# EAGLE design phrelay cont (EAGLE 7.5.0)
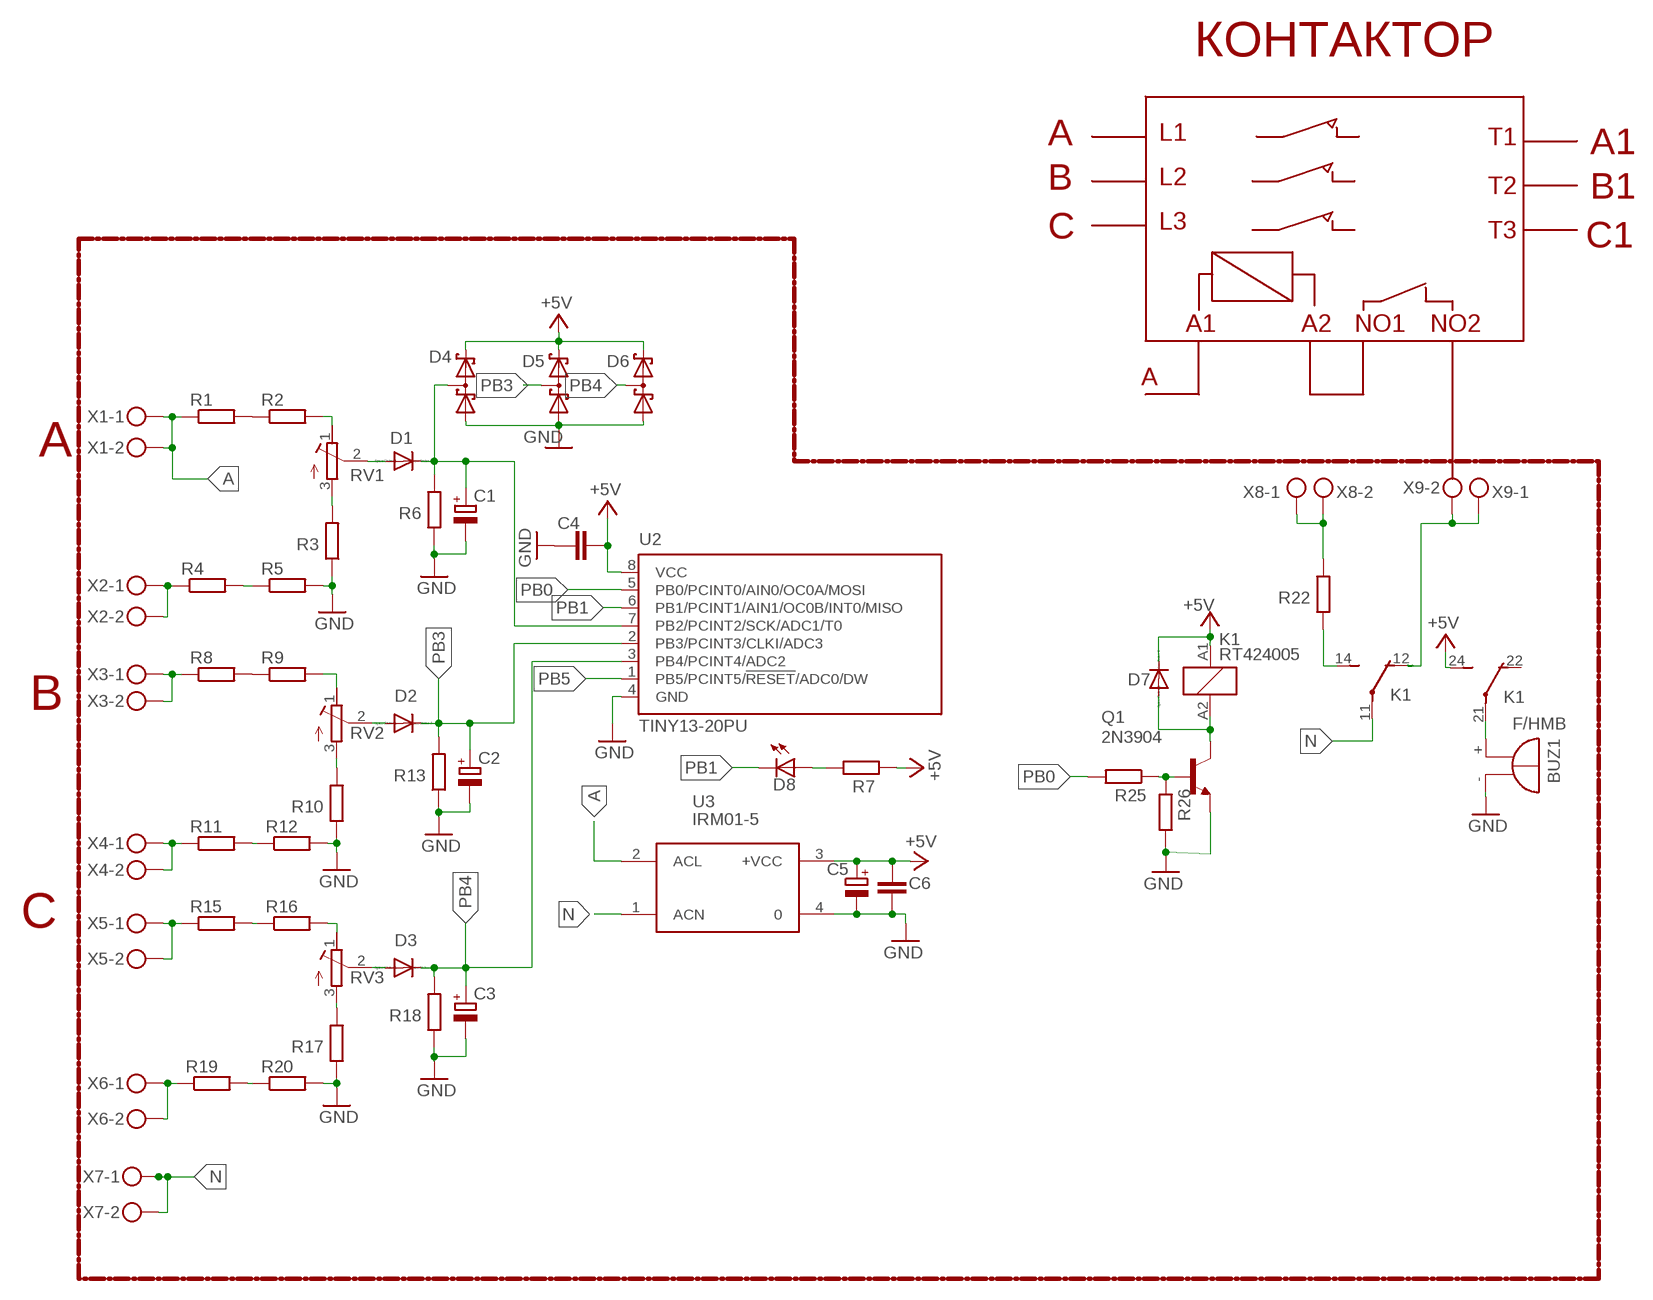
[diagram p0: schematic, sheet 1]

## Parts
BUZ1  F/HMB  [F/HMB]
C1  CPOL-EUE2-5  [E2-5]
C2  CPOL-EUE2-5  [E2-5]
C3  CPOL-EUE2-5  [E2-5]
C4  C-EUC1206  [C1206]
C5  CPOL-EUE2-5  [E2-5]
C6  C-EUC1206  [C1206]
D1  1N4004  [DO41-10]
D2  1N4004  [DO41-10]
D3  1N4004  [DO41-10]
D4  BAT54S  [SOT23]
D5  BAT54S  [SOT23]
D6  BAT54S  [SOT23]
D7  1N4004  [DO41-10]
D8  LED5MM  [LED5MM]
K1  RT424005  [RT2C/O]
Q1  2N3904  [TO92]
R1  R-EU_0414/15  [0414/15]
R2  R-EU_0414/15  [0414/15]
R3  R-EU_0309/12  [0309/12]
R4  R-EU_0414/15  [0414/15]
R5  R-EU_0414/15  [0414/15]
R6  R-EU_R1206  [R1206]
R7  R-EU_R1206  [R1206]
R8  R-EU_0414/15  [0414/15]
R9  R-EU_0414/15  [0414/15]
R10  R-EU_0309/12  [0309/12]
R11  R-EU_0414/15  [0414/15]
R12  R-EU_0414/15  [0414/15]
R13  R-EU_R1206  [R1206]
R15  R-EU_0414/15  [0414/15]
R16  R-EU_0414/15  [0414/15]
R17  R-EU_0309/12  [0309/12]
R18  R-EU_R1206  [R1206]
R19  R-EU_0414/15  [0414/15]
R20  R-EU_0414/15  [0414/15]
R22  R-EU_0309/12  [0309/12]
R25  R-EU_R1206  [R1206]
R26  R-EU_R1206  [R1206]
RV1  R-TRIMM-3386-F  [R-TRIMM-3386F]
RV2  R-TRIMM-3386-F  [R-TRIMM-3386F]
RV3  R-TRIMM-3386-F  [R-TRIMM-3386F]
U2  TINY13-20PU  [DIL08]
U3  IRM01-5  IRM05-2  [IRM05-2]
X1  MKDSN1,5/2-5,08  [MKDSN1,5/2-5,08]
X2  MKDSN1,5/2-5,08  [MKDSN1,5/2-5,08]
X3  MKDSN1,5/2-5,08  [MKDSN1,5/2-5,08]
X4  MKDSN1,5/2-5,08  [MKDSN1,5/2-5,08]
X5  MKDSN1,5/2-5,08  [MKDSN1,5/2-5,08]
X6  MKDSN1,5/2-5,08  [MKDSN1,5/2-5,08]
X7  MKDSN1,5/2-5,08  [MKDSN1,5/2-5,08]
X8  MKDSN1,5/2-5,08  [MKDSN1,5/2-5,08]
X9  MKDSN1,5/2-5,08  [MKDSN1,5/2-5,08]

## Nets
+5V: C4.2 C5.+ C6.2 D4.2(C2) D5.2(C2) D6.2(C2) D7.C K1.24(3:S) K1.A1 R7.1 U2.8(VCC) U3.3(+VCC)
A: R1.1 U3.2(ACL) X1.1 X1.2
GND: BUZ1.- C1.- C2.- C3.- C4.1 C5.- C6.1 D4.1(A1) D5.1(A1) D6.1(A1) Q1.3(E) R3.1 R5.2 R6.1 R10.1 R12.2 R13.1 R17.1 R18.1 R20.2 R26.2 U2.4(GND) U3.4
N: K1.11(2:P) U3.1(ACN) X7.1 X7.2
N$1: R8.2 R9.1
N$2: R2.2 RV1.1(A)
N$3: R1.2 R2.1
N$4: R3.2 RV1.3(E)
N$5: D1.A RV1.2(S)
N$6: C1.+ D1.C D4.3(C1A2) R6.2 U2.7(PB2/PCINT2/SCK/ADC1/T0)
N$7: R4.1 X2.1 X2.2
N$8: R4.2 R5.1
N$9: R19.1 X6.1 X6.2
N$10: R9.2 RV2.1(A)
N$11: R10.2 RV2.3(E)
N$12: D8.A R7.2
N$13: Q1.2(B) R25.1 R26.1
N$14: R11.2 R12.1
N$15: R8.1 X3.1 X3.2
N$16: R17.2 RV3.3(E)
N$17: R16.2 RV3.1(A)
N$18: R15.2 R16.1
N$19: D2.A RV2.2(S)
N$20: D3.A RV3.2(S)
N$21: D7.A K1.A2 Q1.1(C)
N$22: R11.1 X4.1 X4.2
N$23: R19.2 R20.1
N$24: R15.1 X5.1 X5.2
N$25: BUZ1.+ K1.21(3:P)
N$26: R22.2 X8.1 X8.2
N$27: K1.12(2:O) X9.1 X9.2
N$29: K1.14(2:S) R22.1
PB0: R25.2 U2.5(PB0/PCINT0/AIN0/OC0A/MOSI)
PB1: D8.K(C) U2.6(PB1/PCINT1/AIN1/OC0B/INT0/MISO)
PB3: C2.+ D2.C D5.3(C1A2) R13.2 U2.2(PB3/PCINT3/CLKI/ADC3)
PB4: C3.+ D3.C D6.3(C1A2) R18.2 U2.3(PB4/PCINT4/ADC2)
PB5: U2.1(PB5/PCINT5/!RESET!/ADC0/DW)
Unconnected: K1.22(3:O)

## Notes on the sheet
- КОНТАКТОР
- A | L1 | T1
- A1
- B | L2
- T2 | B1
- L3
- C | T3 | C1
- A1 | A2 | NO1 | NO2
- А
- A
- B
- C

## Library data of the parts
BUZ1 = buzzer:F/HMB: BUZZER; OC_FARNELL: unknown; OC_NEWARK: unknown
C1-C3 C5 = rcl:CPOL-EU: POLARIZED CAPACITOR, European symbol
C4 C6 = rcl:C-EU: CAPACITOR, European symbol
D1-D3 D7 = diode:1N4004: DIODE
D4-D6 = diode:BAT54S: Schottky Diodes Pin connection corrected 2011-05-04 Source: Fairchild .. BAT54.pdf
D8 = led:LED: LED
K1 = relay:RT42?*: Power PCB Relay SCHRACK 2 pole 8 A, DC and AC-coil Source: http://www.schrack.com/.. 5842.pdf; MPN: RT424005; OC_FARNELL: 1629052; OC_NEWARK: 03P2425
Q1 = transistor:2N3904: NPN TRANSISTOR
R1-R13 R15-R20 R22 R25 R26 = rcl:R-EU_: RESISTOR, European symbol
RV1-RV3 = rcl:R-TRIMM-3386-F
U2 = atmel:TINY13: 8-bit AVR Microcontroller with 1K Bytes In-System Programmable Flash Source: http://www.atmel.com/dyn/resources/prod_documents/2535S.pdf; MPN: ATTINY13-20PU; OC_FARNELL: 9171550; OC_NEWARK: 96K6521
U3 = acdc:IRM05-2
X1-X9 = con-phoenix-508:MKDSN1,5/2-5,08: MKDSN 1,5/ 2-5,08 Printklemme

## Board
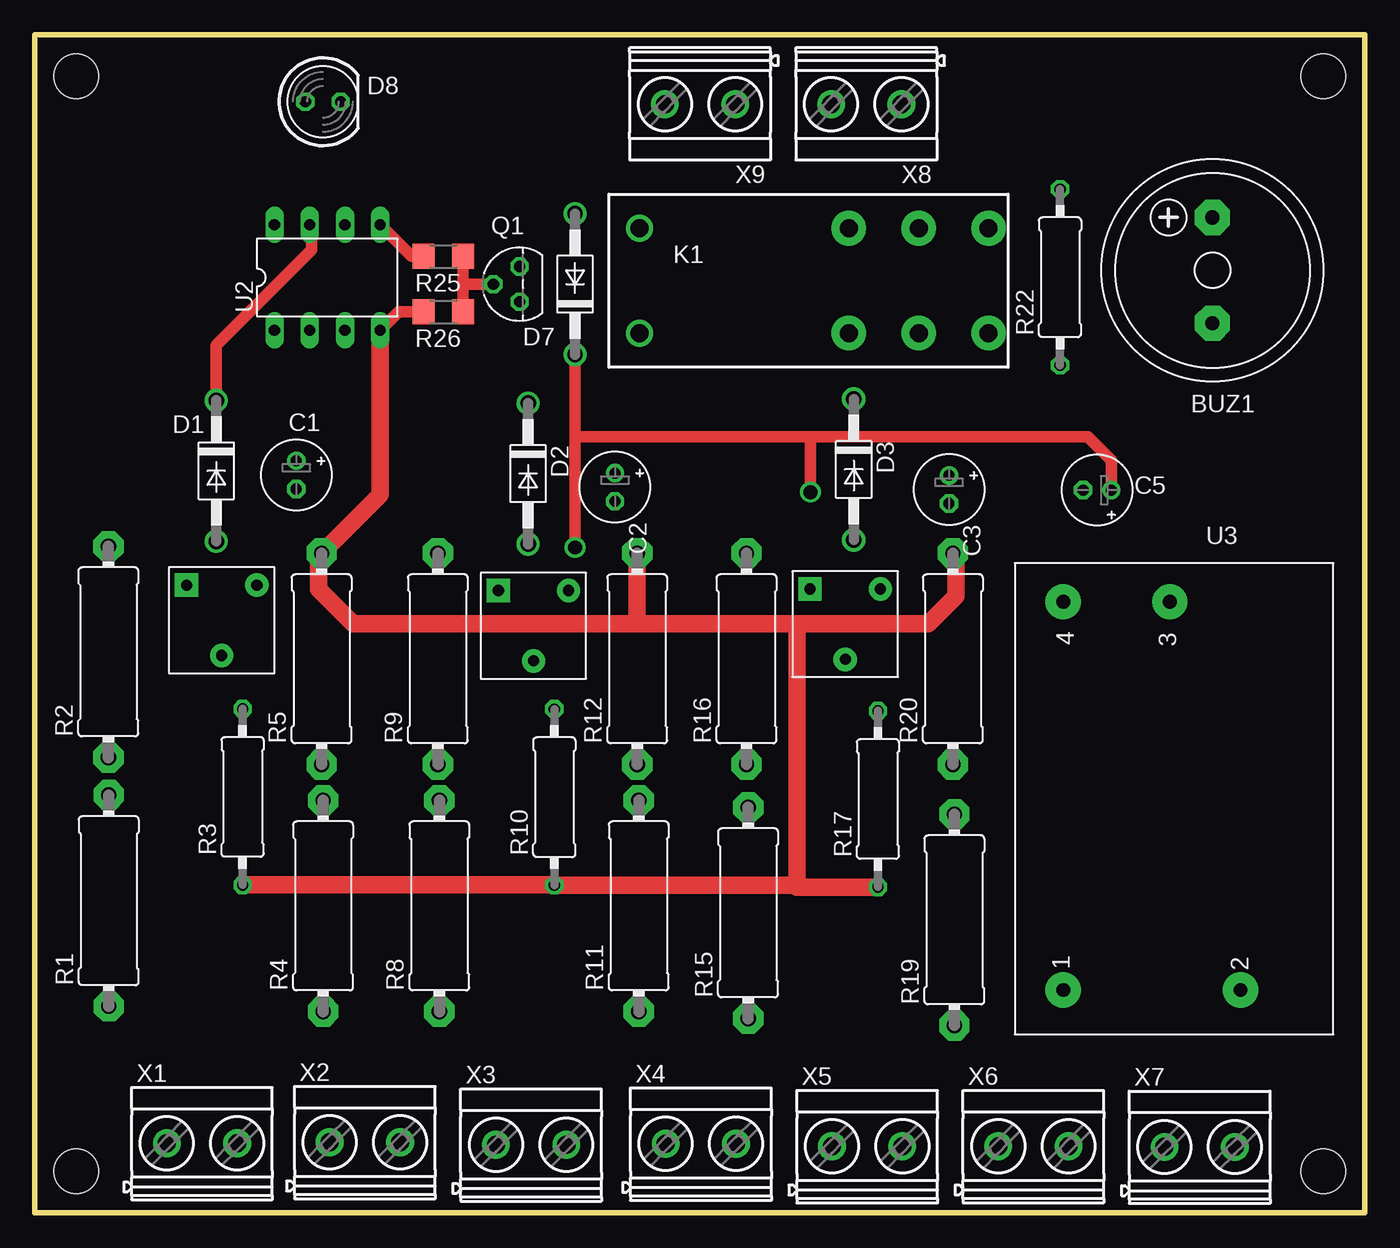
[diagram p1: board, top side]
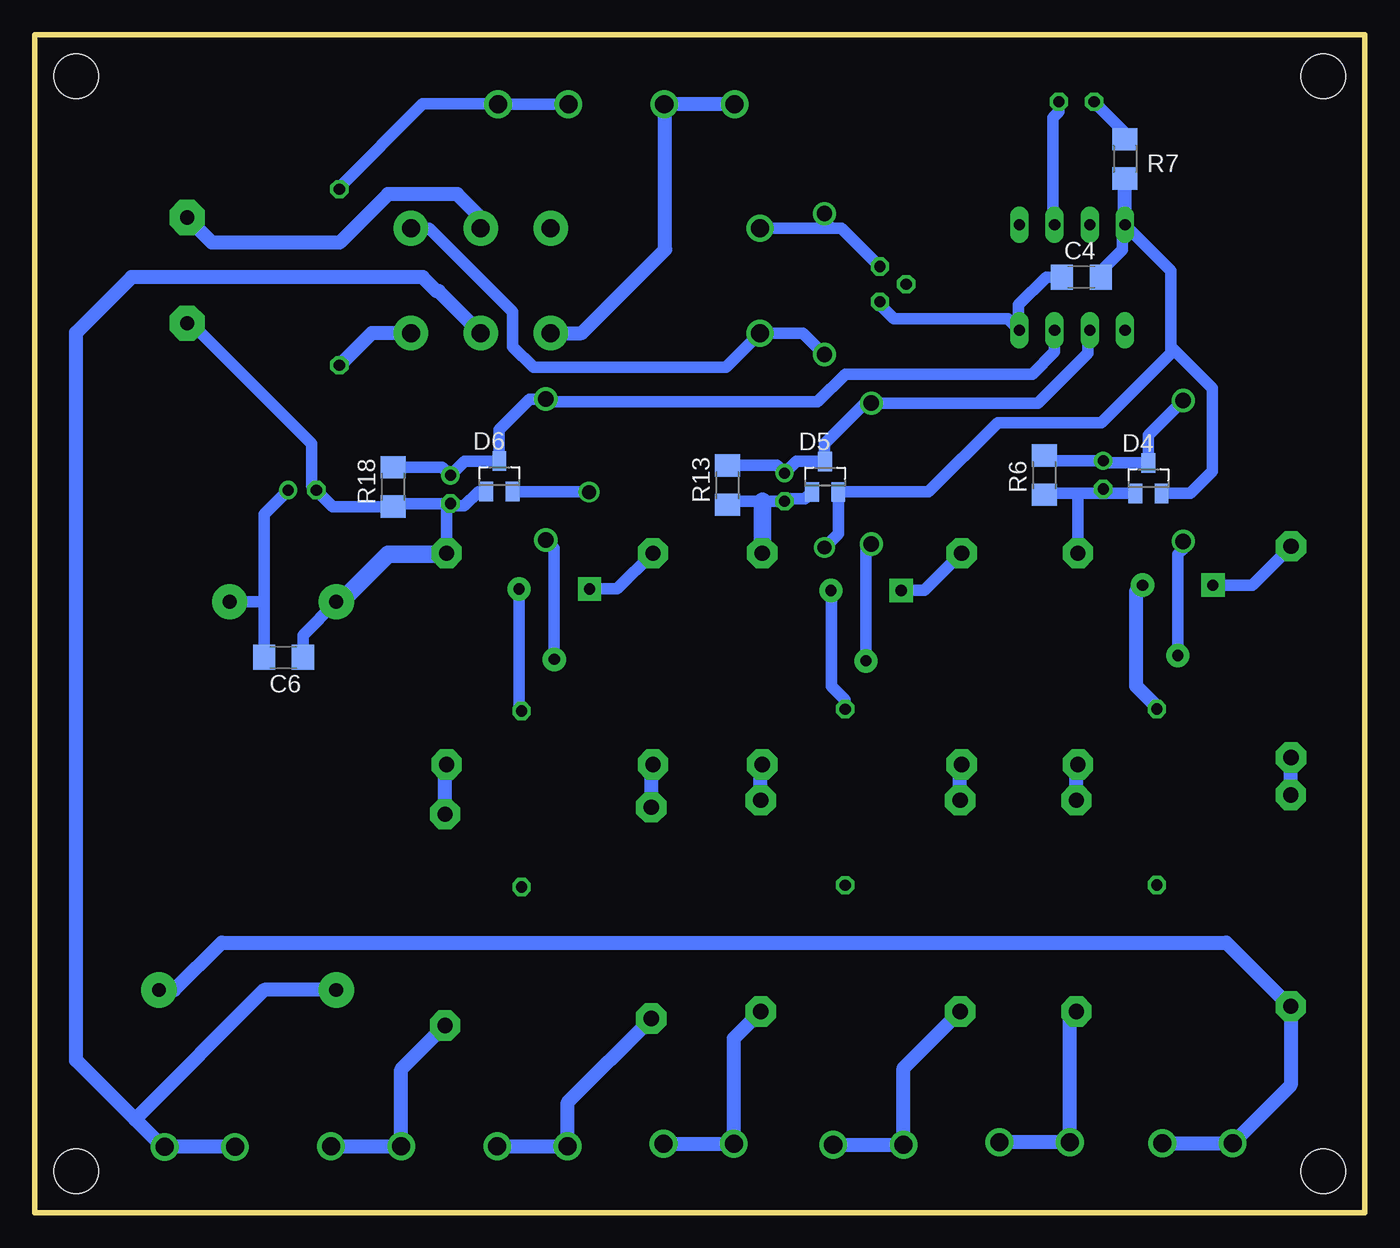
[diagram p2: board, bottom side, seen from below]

Size 96 x 85 mm. Coordinates in mm from the lower left corner, seen from the top.
Outline: 0,0 96,0 96,85 0,85 0,0
Copper layers (1*16): Top 0.035mm / dielectric 1.5mm / Bottom 0.035mm
Design rules "default": minimum track width 10mil, minimum drill 24mil, track to track 8mil, track to pad 8mil, pad to pad 8mil, via to via 8mil, smd to smd 8mil, copper to edge 40mil, drill to drill 8mil, minimum pad ring 10mil, minimum via ring 8mil, stop-mask expansion 4mil, vias tented up to drill 0mil, thermal gap 10mil
Holes 3.2 mm at 3,3 93,3 3,82 93,82

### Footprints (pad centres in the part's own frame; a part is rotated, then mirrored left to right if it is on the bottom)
F/HMB = drill 1.016 pad 2.54 octagon: + 3.81,0; - -3.81,0
E2-5 = drill 0.813 pad 1.27: + -1.016,0 | drill 0.813 pad 1.27 octagon: - 1.016,0
C1206 = smd 1.6 x 1.8: 1 -1.4,0; 2 1.4,0
DO41-10 = drill 1.118: A 5.08,0; C -5.08,0
SOT23 = smd 1 x 1.4: 1 -0.95,-1.1; 2 0.95,-1.1; 3 0,1.1
LED5MM = drill 0.813 octagon: A -1.27,0; K 1.27,0
RT2C/O = drill 1.3 pad 2.5: 11 7.56,-3.68; 12 2.52,-3.68; 14 12.6,-3.68; 21 7.56,3.88; 22 2.52,3.88; 24 12.6,3.88 | drill 1.3: A1 -12.6,-3.68; A2 -12.6,3.88
TO92 = drill 0.813 octagon: 1 1.27,0; 2 0,1.905; 3 -1.27,0
0414/15 = drill 1.1 pad 2.184 octagon: 1 -7.62,0; 2 7.62,0
0309/12 = drill 0.813 octagon: 1 -6.35,0; 2 6.35,0
R1206 = smd 1.6 x 1.803: 1 -1.422,0; 2 1.422,0
R-TRIMM-3386F = drill 0.8 pad 1.676 square: 1 0,0 | drill 0.8 pad 1.676: 2 5.08,2.54; 3 0,5.08
DIL08 = drill 0.813 long: 1 -3.81,-3.81; 2 -1.27,-3.81; 3 1.27,-3.81; 4 3.81,-3.81; 5 3.81,3.81; 6 1.27,3.81; 7 -1.27,3.81; 8 -3.81,3.81
IRM05-2 = drill 1 pad 2.54: 1 30.8,3.5; 2 30.8,16.3; 3 2.8,11.2; 4 2.8,3.5
MKDSN1,5/2-5,08 = drill 1.3 pad 2: 1 -2.561,0.025; 2 2.519,0.025

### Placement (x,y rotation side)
BUZ1  85,68 90 top
C1  18.88,53.24 270 top
C2  41.88,52.35 270 top
C3  65.99,52.19 270 top
C4  20.46,67.51 0 bottom
C5  76.69,52.14 180 top
C6  78.04,40.07 180 bottom
D1  13.11,53.53 270 top
D2  35.61,53.33 270 top
D3  59.11,53.63 270 top
D4  15.62,53 0 bottom
D5  38.96,53.11 0 bottom
D6  62.46,53.14 0 bottom
D7  39,67 90 top
D8  20.81,80.16 0 top
K1  56.24,67.15 0 top
Q1  35,67 90 top
R1  5.35,22.52 90 top
R2  5.32,40.47 90 top
R3  15.01,30.01 90 top
R4  20.82,22.14 90 top
R5  20.71,39.97 90 top
R6  23.14,53.22 90 bottom
R7  17.31,76.04 90 bottom
R8  29.21,22.14 90 top
R9  29.1,39.97 90 top
R10  37.51,29.99 90 top
R11  43.6,22.14 90 top
R12  43.49,39.97 90 top
R13  46,52.5 90 bottom
R15  51.49,21.64 90 top
R16  51.38,39.97 90 top
R17  60.86,29.86 90 top
R18  70.14,52.38 90 bottom
R19  66.38,21.14 90 top
R20  66.27,39.97 90 top
R22  74,67.5 90 top
R25  29.5,69 180 top
R26  29.5,65 180 top
RV1  10.96,45.29 270 top
RV2  33.46,44.9 270 top
RV3  55.96,45.01 270 top
U2  21.12,67.48 0 top
U3  70.73,46.88 270 top
X1  12.1,5 0 top
X2  23.85,5.07 0 top
X3  35.85,4.89 0 top
X4  48.1,4.96 0 top
X5  60.1,4.78 0 top
X6  72.1,4.78 0 top
X7  84.1,4.73 0 top
X8  60,80 180 top
X9  48,80 180 top

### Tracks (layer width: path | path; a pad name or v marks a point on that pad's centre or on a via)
+5V  (via drill 1)
  Top 0.813: D7.C 39,56 | 39,56 v39,48 | C5.+ 77.71,54.29 76,56 56,56 | 56,56 39,56 | v56,52 56,56
  Bottom 0.813: C6.2 79.44,44 | 79.44,44 79.44,50.41 C5.+ | U3.3 79.52,44.08 79.44,44 | D5.2 37.99,52.01 | 14,62.5 14,62 19,57 26.5,57 31.49,52.01 D5.2 | 14,62.5 14,67.98 U2.8 17.5,71.1 17.5,69.5 19.06,67.94 C4.2 | D4.2 12.6,51.9 11,53.5 11,59.5 14,62.5 | v39,48 38,49 D5.2 | D7.C 40.55,63.47 K1.A1 46.11,61 60,61 61.5,62.5 61.5,65 67.53,71.03 K1.24 | D6.2 56.04,52.04 v56,52
  Bottom 1.016: U2.8 R7.1
A
  Bottom 1.016: X1.2 X1.1 5.35,9.21 R1.1 5.95,15.5 6,15.5 10,19.5 82.5,19.5 85.92,16.08 U3.2
GND
  Top 0.813: R26.2 26.26,65 U2.4
  Top 1.27: 55,42.5 64.5,42.5 66.5,44.5 66.5,47.36 R20.2 | 55,42.5 43.5,42.5 | 43.5,42.5 23,42.5 20.5,45 20.5,47.38 R5.2 24.93,51.81 U2.4 | 55,23.5 55,42.5 | R3.1 37.49,23.66 R10.1 54.86,23.64 55,23.5 | R12.2 43.49,42.51 43.5,42.5 | 55,23.5 R17.1
  Bottom 0.813: D4.1 18.5,51.9 | 18.5,51.9 20.5,51.9 | 20.5,51.9 23.04,51.9 R6.1 | C1.- 18.82,52.22 18.5,51.9 | R5.2 20.71,51.69 20.5,51.9 | 43.5,51.33 C2.- 41.7,51.51 40.41,51.51 D5.1 | 43.5,51.33 45.74,51.33 R13.1 | R20.2 66.27,50.89 C3.- | C3.- 69.92,51.17 R18.1 74.49,50.96 C5.- 76,52.47 76,55.5 84.69,64.19 BUZ1.- | D6.1 63.96,52.04 65,51 65.82,51 C3.- | 43.49,51.32 43.5,51.33 | C4.1 22.99,67.51 25,65.5 25,63.74 U2.4 25.76,64.5 34,64.5 35,65.5 Q1.3 | C6.1 76.64,41.67 U3.4
  Bottom 1.016: 37.49,23.66 R10.1
  Bottom 1.27: R12.2 43.49,51.32 | U3.4 73.92,44.08 70.5,47.5 66.36,47.5 R20.2
N
  Bottom 1.016: 88.75,6.75 86.75,4.75 X7.2 X7.1 | 88.75,6.75 93,11 93,63.5 89,67.5 68,67.5 67,66.5 66.83,66.5 K1.11 | U3.1 79.42,16.08 88.75,6.75
N$1
  Bottom 1.016: R8.2 29.21,32.24 R9.1
N$2
  Bottom 0.813: RV1.1 8.12,45.29 R2.2
N$3
  Bottom 1.016: R1.2 5.35,32.82 R2.1
N$4
  Bottom 1.016: R3.2 15.01,36.51 16.5,38 16.5,44.83 RV1.3
N$5
  Bottom 0.813: D1.A 13.11,47.89 13.5,47.5 RV1.2
N$6
  Top 0.813: D1.C 13.11,62.61 20,69.5 20,71.14 U2.7
  Bottom 0.813: D1.C 15.62,56.1 D4.3 18.72,54.1 C1.+ 22.75,54.26 R6.2
N$7
  Bottom 1.016: R4.1 21.29,14.05 X2.1 X2.2
N$8
  Bottom 1.016: R4.2 20.82,32.24 R5.1
N$9
  Bottom 1.016: X6.2 X6.1 69.54,10.36 R19.1
N$10
  Bottom 0.813: RV2.1 31.79,44.9 R9.2
N$11
  Bottom 0.813: R10.2 37.51,37.01 38.5,38 38.5,44.86 RV2.3
N$12
  Bottom 0.813: R7.2 17.31,77.93 D8.A
N$13
  Top 0.813: R26.1 30.92,67 | 30.92,67 R25.1 | Q1.2 30.92,67
N$14
  Bottom 1.016: R11.2 43.6,32.24 R12.1
N$15
  Bottom 1.016: X3.2 X3.1 33.29,10.44 R8.1
N$16
  Bottom 0.813: RV3.3 61.04,36.39 R17.2
N$17
  Bottom 0.813: RV3.1 53.96,45.01 R16.2
N$18
  Bottom 1.016: R15.2 51.49,32.24 R16.1
N$19
  Bottom 0.813: RV2.2 36,47.86 D2.A
N$20
  Bottom 0.813: RV3.2 58.5,47.94 D3.A
N$21
  Bottom 0.813: K1.A2 38.5,71.03 | 38.5,71.03 37.76,71.03 Q1.1 | D7.A 39,71.53 38.5,71.03
N$22
  Bottom 1.016: X4.2 X4.1 45.54,12.58 R11.1
N$23
  Bottom 1.016: R19.2 66.38,32.24 R20.1
N$24
  Bottom 1.016: X5.2 X5.1 57.54,7.97 R15.1
N$25
  Bottom 1.016: K1.21 63.8,71.8 65.5,73.5 70.5,73.5 74,70 83.19,70 BUZ1.+
N$26
  Bottom 0.813: X8.2 X8.1 62.59,80 68,80 74,74 R22.2
N$27
  Bottom 1.016: K1.12 56.53,63.47 50.5,69.5 50.5,79.91 X9.1 X9.2
N$29
  Bottom 1.016: K1.14 71.68,63.47 R22.1
PB0
  Top 0.813: R25.2 27.22,69 U2.5
PB1
  Bottom 0.813: D8.K 22.08,79.42 22.5,79 22.5,71.4 U2.6
PB3
  Bottom 0.813: R13.2 42.44,53.92 C2.+ 41.04,54.21 D5.3 39,54.25 39,55.5 36.09,58.41 D2.C 23.59,58.41 20,62 20,63.52 U2.2
PB4
  Bottom 0.813: R18.2 66.59,53.8 C3.+ 64.96,54.24 D6.3 62.5,54.28 62.5,56.5 60.29,58.71 D3.C 58.9,58.5 39.5,58.5 37.5,60.5 24,60.5 22.39,62.11 U2.3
